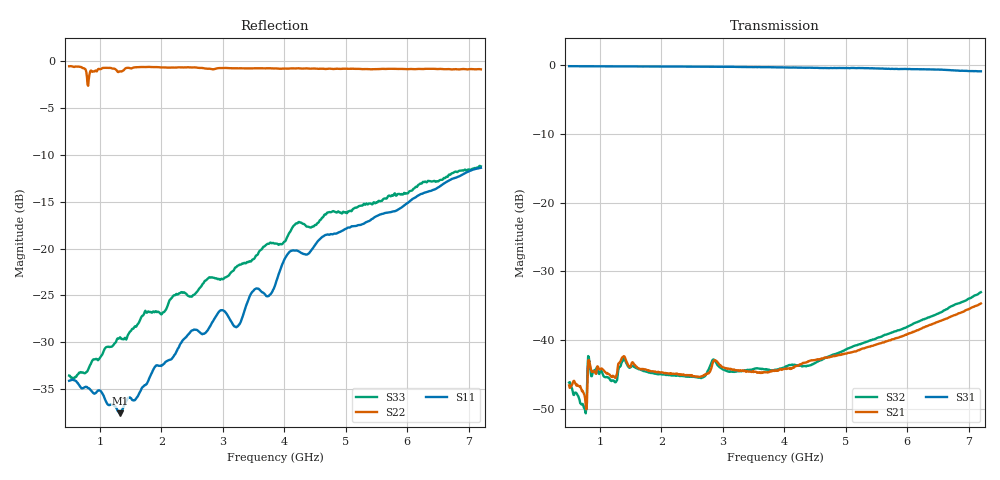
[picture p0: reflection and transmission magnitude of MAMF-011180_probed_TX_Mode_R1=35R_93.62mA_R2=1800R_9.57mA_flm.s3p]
! MAMF-011180 Probed Data: no bias components
! TX Mode
!  Port 1 =  ANT
!  Port 2 =  RX
!  Port 3 =  TX
! This data represents a typical device, and is provided for engineering reference only.
! This data does not change MACOM's datasheet specifications.
! For questions on this and other MACOM Components, please visit MACOM.com and click on support.
! Technical support requests go to MACOM's application engineering team.
# Hz S  dB  R 50
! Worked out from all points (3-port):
!   671 points, 500 MHz to 7.2 GHz, reference 50 ohm
!   strongest paths, dB at 500 MHz, 2.17 GHz, 3.85 GHz, 5.53 GHz, 7.2 GHz:
!     S31: -0.2, -0.2, -0.3, -0.5, -0.9
!     S21: -46.6, -44.9, -44.4, -40.6, -34.7
!     S32: -46.2, -45.2, -44.3, -39.6, -33.0
!   lowest |S11| = -37.6 dB at 1.33 GHz (marker M1), VSWR 1.03, Z = 50.3 - j1.29 ohm
!   |S11| at or under -10 dB: start of sweep to end of sweep
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5e8  -34.10 -18.6  -46.64 10.8  -0.17 -8.8
     -46.58 10.4  -0.54 -168.0  -46.13 8.6
     -0.16 -8.8  -46.17 8.2  -33.55 -17.3
7.5e8  -34.80 -31.6  -47.94 14.4  -0.18 -13.1
       -47.99 15.0  -0.80 177.6  -49.93 22.6
       -0.18 -13.1  -49.92 23.0  -33.31 -22.9
8.3e8  -34.95 -39.1  -43.11 23.5  -0.18 -14.5
       -43.13 23.8  -1.44 -176.4  -43.13 19.9
       -0.18 -14.5  -43.10 19.7  -32.58 -26.1
1.24e9  -36.82 -62.8  -45.44 13.7  -0.19 -21.6
        -45.38 14.3  -0.80 168.9  -46.03 10.7
        -0.19 -21.5  -46.08 10.5  -30.11 -39.1
1.33e9  -37.58 -76.5  -43.19 17.1  -0.20 -23.1
        -43.19 17.1  -1.08 168.6  -43.85 15.3
        -0.20 -23.1  -43.86 15.4  -29.46 -39.5
2.5e9  -28.74 -146.3  -45.17 0.8  -0.23 -43.6
       -45.09 0.7  -0.67 145.8  -45.29 -5.3
       -0.24 -43.6  -45.33 -5.3  -25.12 -75.2
3.85e9  -23.94 154.0  -44.46 5.2  -0.33 -67.7
        -44.43 5.6  -0.77 124.6  -44.31 -9.6
        -0.32 -67.7  -44.32 -9.3  -19.46 -102.8
4.1e9  -20.29 155.5  -44.13 7.1  -0.38 -72.2
       -44.20 6.7  -0.76 120.0  -43.63 -7.8
       -0.35 -72.3  -43.63 -7.9  -18.17 -102.0
5.65e9  -16.19 135.9  -40.23 10.0  -0.51 -101.3
        -40.19 9.9  -0.83 97.3  -39.20 -7.8
        -0.53 -101.4  -39.21 -7.8  -14.65 -150.7
7.2e9  -11.38 115.8  -34.76 0.5  -0.92 -134.6
       -34.68 1.3  -0.87 76.1  -32.97 -26.8
       -0.91 -133.9  -33.03 -26.6  -11.22 155.8
